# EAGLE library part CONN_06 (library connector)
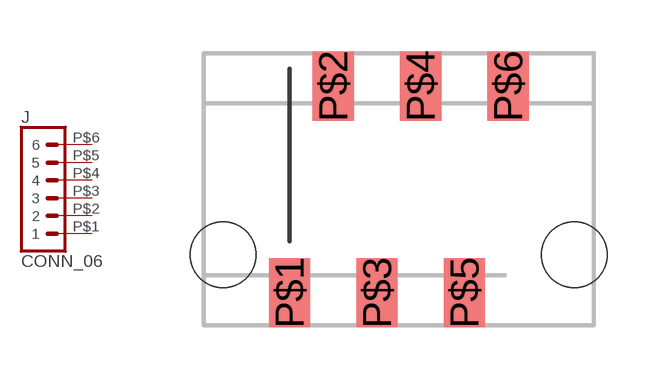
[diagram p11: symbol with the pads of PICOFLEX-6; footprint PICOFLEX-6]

Designator prefix J

## CONN_06PICOFLEX  [PICOFLEX-6]
P$1  1  pas
P$2  2  pas
P$3  3  pas
P$4  4  pas
P$5  5  pas
P$6  6  pas

## Footprint PICOFLEX-6 (pad centres in mm)
smd 1.2 x 2: P$1 0,0; P$2 1.27,6; P$3 2.54,0; P$4 3.81,6; P$5 5.08,0; P$6 6.35,6
hole 1.9 at -1.93,1.1
hole 1.9 at 8.27,1.1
